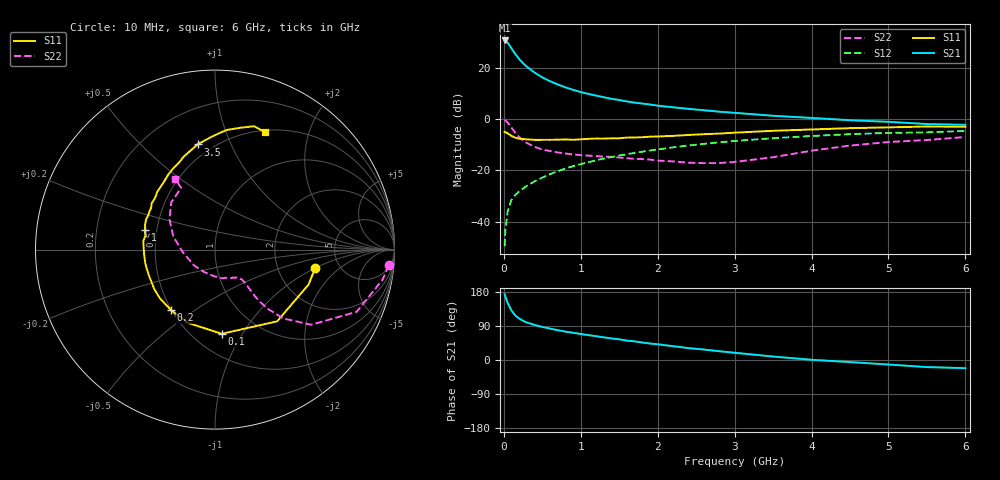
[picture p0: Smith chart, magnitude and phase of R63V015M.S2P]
! SIEMENS Small Signal Semiconductors
! BFR193
! Si NPN RF Bipolar Junction Transistor in SOT23
! VCE = 3 V  IC = 15 mA
! Common Emitter S-Parameters:  May  1996
# GHz  S  MA  R  50
!  f  S11  S21  S12  S22
! GHz  MAG  ANG  MAG  ANG  MAG  ANG  MAG  ANG
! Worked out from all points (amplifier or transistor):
!   36 points, 10 MHz to 6 GHz, reference 50 ohm
!   highest |S21| = 30.8 dB at 10 MHz (marker M1)
!   |S21| within 3 dB of that: start of sweep to 96.78 MHz
!   unconditionally stable (mu >= 1): 633.9 MHz to 1.878 GHz; 1.96 GHz to 2.019 GHz
!   at 250 MHz: K = 0.76, MSG = 24.5 dB, |S12| = -27.1 dB
!   at 1.4 GHz: K = 1.03, MAG = 10.3 dB, |S12| = -14.8 dB
!   at 6 GHz: K = 0.94, MSG = 1.2 dB, |S12| = -4.6 dB
!   S11 on the Smith chart (normalised r, x): 10 MHz: 3.29, -1.00; 100 MHz: 0.68, -0.82; 200 MHz: 0.50, -0.40; 1 GHz: 0.43, +0.11; 3.5 GHz: 0.42, +0.76; 6 GHz: 0.53, +1.38
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0.01  0.5675 -10.5  34.65 173.6  0.0033 88.3  0.9719 -5.1
0.02  0.5565 -20.5  34.34 167.1  0.0067 83.4  0.9491 -10.1
0.05  0.5287 -49.1  31.24 150.4  0.0159 72.3  0.8622 -23.7
0.1  0.4708 -85.4  24.12 130.4  0.0268 63.2  0.6801 -38.0
0.15  0.4352 -110.4  18.75 117.3  0.0333 59.7  0.539 -45.3
0.2  0.4166 -126.1  15.02 109.3  0.0389 60.1  0.4467 -48.1
0.25  0.4101 -138.2  12.39 103.4  0.0443 60.5  0.386 -49.3
0.3  0.4037 -146.9  10.58 98.9  0.05 61.9  0.3429 -49.4
0.4  0.3954 -159.7  8.147 92.6  0.0609 63.8  0.2882 -48.7
0.5  0.3958 -168.6  6.567 87.3  0.0722 65.5  0.2552 -47.8
0.6  0.3957 -175.5  5.532 82.9  0.0842 66.1  0.2395 -48.1
0.7  0.3975 178.8  4.788 78.6  0.0962 66.4  0.2245 -47.9
0.8  0.4023 173.3  4.202 74.9  0.1083 66.2  0.2138 -49.3
1  0.405 164.1  3.394 68.6  0.1328 65.6  0.1988 -50.7
1.1  0.4134 160.5  3.119 65.7  0.1449 65.0  0.1941 -53.3
1.4  0.4234 149.3  2.501 56.8  0.182 62.6  0.184 -59.8
1.6  0.4376 143.7  2.227 51.1  0.2071 60.3  0.1726 -65.8
2.2  0.4724 127.1  1.71 36.4  0.2819 53.2  0.1498 -90.6
3.5  0.5941 99.4  1.168 9.1  0.4252 34.0  0.1807 -175.8
4.5  0.669 84.6  0.956 -5.5  0.5104 19.5  0.3053 146.2
5.5  0.7213 72.4  0.805 -18.7  0.553 4.7  0.3923 118.7
6  0.7104 66.7  0.776 -21.5  0.5901 0.4  0.4491 119.4
